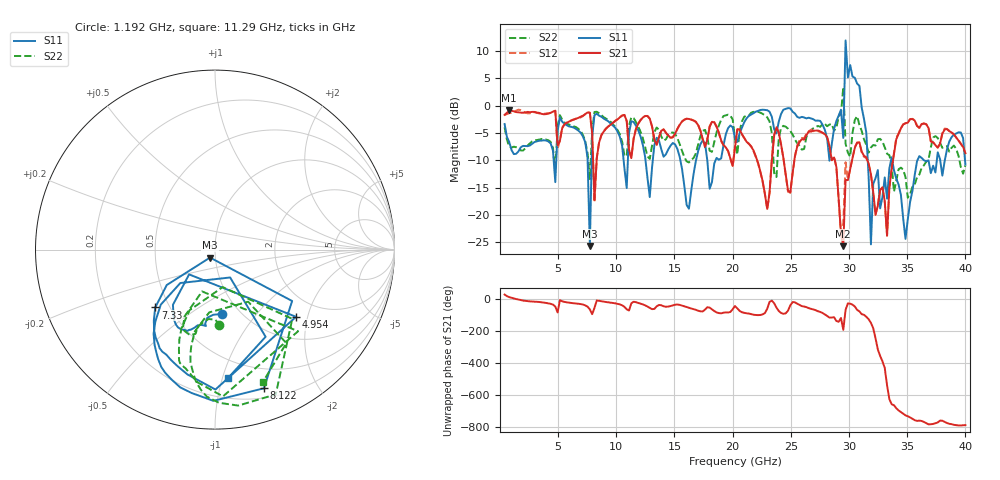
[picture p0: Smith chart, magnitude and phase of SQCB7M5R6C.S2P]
! Network Analyzer HP8722ES.07.66: Jul 25, 2000 Serial No. US39175408
! 26 Oct 2004  15:31:42
! Frequency  S11  S21  S12  S22
# HZ  S  DB R  50
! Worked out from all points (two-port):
!   201 points, 400 MHz to 40 GHz, reference 50 ohm
!   highest |S21| = -0.85 dB at 796 MHz (marker M1); lowest = -25.7 dB at 29.51 GHz (marker M2)
!   |S21| within 3 dB of the highest: start of sweep to 4.848 GHz; 5.418 GHz to 7.862 GHz (2.444 GHz wide, 36.8 % of centre)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
!   lowest |S11| = -25.6 dB at 7.726 GHz (marker M3), VSWR 1.11, Z = 47.1 - j4.2 ohm
!   |S11| at or under -10 dB: 15.51 GHz to 16.85 GHz (1.345 GHz wide, 8.31 % of centre); 31.61 GHz to 33.61 GHz (1.999 GHz wide, 6.13 % of centre); 33.71 GHz to 35.88 GHz (2.165 GHz wide, 6.22 % of centre)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
!   |S22| runs from -16.8 to 3.4 dB; largest |S21 - S12| = 0.14
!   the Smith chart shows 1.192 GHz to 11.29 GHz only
!   S11 on the Smith chart (normalised r, x): 1.192 GHz: 0.83, -0.68; 4.954 GHz: 1.49, -1.70; 7.33 GHz: 0.42, -0.34; 8.122 GHz: 0.29, -1.37; 11.29 GHz: 0.35, -1.04
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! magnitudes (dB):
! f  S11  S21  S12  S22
! 400 MHz  -3.4  -1.7  -1.7  -4.0
! 796 MHz  -6.6  -0.9  -1.4  -7.5
! 1.192 GHz  -8.9  -1.0  -1.2  -7.5
! 4.954 GHz  -4.6  -7.2  -7.9  -3.8
! 7.132 GHz  -5.6  -1.8  -1.9  -5.4
! 7.33 GHz  -6.7  -1.6  -1.6  -6.5
! 7.726 GHz  -25.6  -1.3  -1.3  -13.4
! 8.122 GHz  -1.7  -17.3  -17.7  -1.2
! 10.89 GHz  -15.1  -2.8  -2.9  -9.3
! 11.29 GHz  -2.8  -9.6  -9.5  -2.1
! 13.67 GHz  -6.4  -5.8  -5.7  -4.4
! 16.24 GHz  -18.8  -2.4  -2.4  -10.4
! 20.2 GHz  -5.9  -7.7  -7.4  -6.1
! 22.97 GHz  -0.8  -18.9  -19.0  -2.1
! 26.93 GHz  -2.5  -4.6  -4.7  -4.1
! 29.51 GHz  -5.9  -25.7  -21.6  3.4
! 29.7 GHz  11.9  -13.6  -10.4  -7.0
! 31.49 GHz  -5.0  -9.4  -9.6  -7.2
! 31.88 GHz  -25.4  -12.5  -12.6  -7.6
! 33.47 GHz  -11.5  -15.0  -14.9  -9.1
! 34.85 GHz  -24.4  -3.2  -3.2  -13.1
! 40 GHz  -10.8  -8.7  -8.8  -10.9
